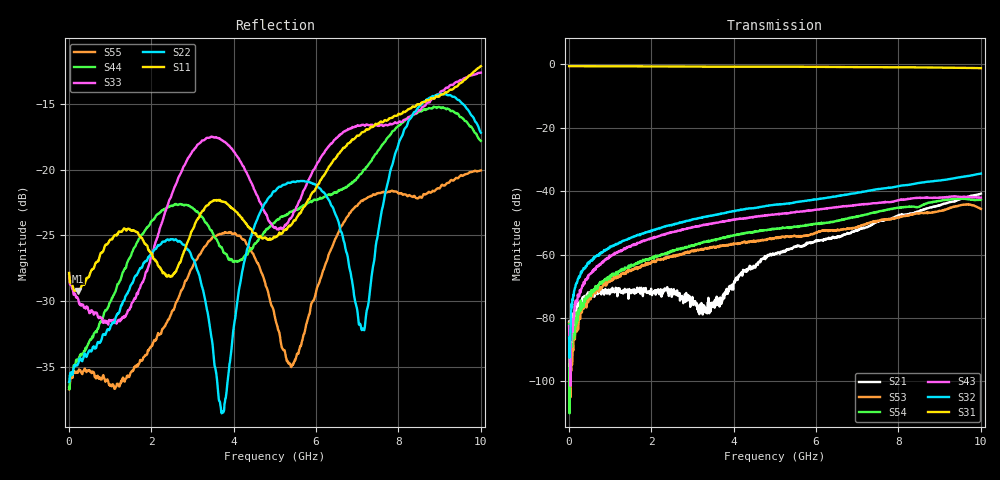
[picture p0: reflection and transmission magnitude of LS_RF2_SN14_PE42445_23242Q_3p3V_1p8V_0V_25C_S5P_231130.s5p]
!Keysight Technologies,M9804A,MY58100185,A.15.10.06
!Date: Thursday, November 30, 2023 12:04:37
!Correction: S11(Cdelta 6-Port  )
!S12(Cdelta 6-Port  )
!S13(Cdelta 6-Port  )
!S15(Cdelta 6-Port  )
!S16(Cdelta 6-Port  )
!S21(Cdelta 6-Port  )
!S22(Cdelta 6-Port  )
!S23(Cdelta 6-Port  )
!S25(Cdelta 6-Port  )
!S26(Cdelta 6-Port  )
!S31(Cdelta 6-Port  )
!S32(Cdelta 6-Port  )
!S33(Cdelta 6-Port  )
!S35(Cdelta 6-Port  )
!S36(Cdelta 6-Port  )
!S51(Cdelta 6-Port  )
!S52(Cdelta 6-Port  )
!S53(Cdelta 6-Port  )
!S55(Cdelta 6-Port  )
!S56(Cdelta 6-Port  )
!S61(Cdelta 6-Port  )
!S62(Cdelta 6-Port  )
!S63(Cdelta 6-Port  )
!S65(Cdelta 6-Port  )
!S66(Cdelta 6-Port  )
!S5P File: Measurements: <S11,S12,S13,S15,S16>,
!<S21,S22,S23,S25,S26>,
!<S31,S32,S33,S35,S36>,
!<S51,S52,S53,S55,S56>,
!<S61,S62,S63,S65,S66>:
# Hz S  dB  R 50
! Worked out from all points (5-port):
!   1000 points, 10 MHz to 10 GHz, reference 50 ohm
!   strongest paths, dB at 10 MHz, 2.51 GHz, 5.01 GHz, 7.51 GHz, 10 GHz:
!     S31: -0.6, -0.7, -0.7, -0.9, -1.2
!     S32: -86.2, -50.6, -44.3, -39.3, -34.5
!     S43: -82.6, -52.9, -47.4, -43.7, -42.0
!     S54: -82.0, -58.8, -51.9, -46.5, -42.7
!     S53: -81.5, -60.6, -54.8, -49.4, -45.6
!     S21: -81.2, -72.7, -59.9, -49.7, -40.8
!   lowest |S11| = -29.2 dB at 220 MHz (marker M1), VSWR 1.07, Z = 53.1 - j1.68 ohm
!   |S11| at or under -10 dB: start of sweep to end of sweep
